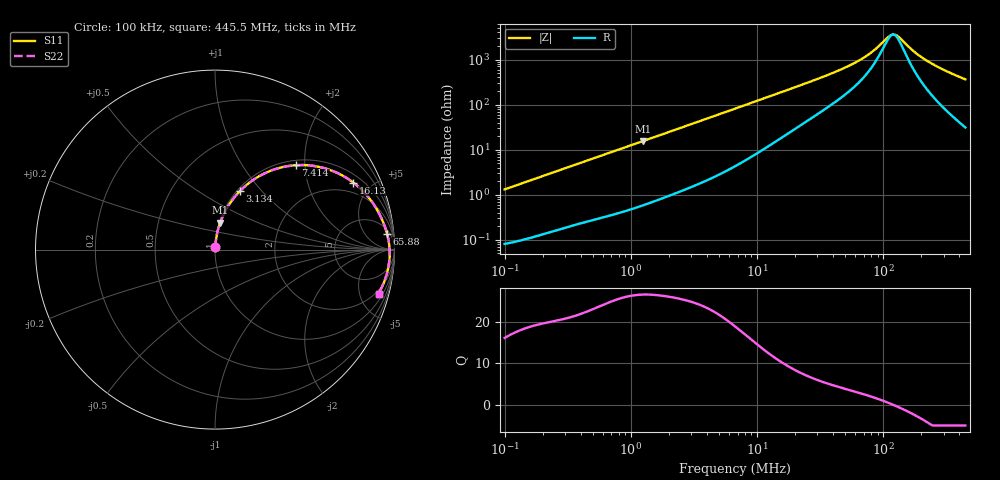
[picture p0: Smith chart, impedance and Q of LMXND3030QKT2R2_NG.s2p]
! LMXND3030QKT2R2_NG  S-PARAMETER MODEL  ( General Type )
! Model Generated by TAIYO YUDEN Corporation (http://www.ty-top.com)
! Version 1.0
! TAIYO YUDEN Control No. 191023NI43SB-FBB
! Copyright(c) 2019 TAIYO YUDEN CO.,LTD. All Rights Reserved.
! Product Description (link to TY-COMPAS)
! https://ds.yuden.co.jp/TYCOMPAS/or/detail?pn=LMXND3030QKT2R2MNG&u=M
! Products Name : Inductors
! Characteristics :
!  Inductance : 2.2 uH , SRF(min) : 64 MHz , DC Resistance(max) : 0.0696 Ohm
!  Rated Current : Saturation :1480 mA , Temp Rise : 1500 mA
!  Case Size : 3.0 x 3.0 / 0.118 x 0.118 [mm/inch] , Thickness : 1.5 / 0.059 [mm/inch]
!  (Conditions: Temperature = 25 degC , DC Bias Current/Voltage = 0A / 0V)
! External Node Assignments :
!  1  o---GGG---o  2
! GND o---------o GND
! Frequency Range : 0.1MHz  -  445.549718MHz  [ 402 STEP ]
# MHz S RI R 50
! Freq[MHz].  S11 Real  S11 Imag  S21 Real  S21 Imag  S12 Real  S12 Imag  S22 Real  S22 Imag
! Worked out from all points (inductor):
!   401 points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, 100 kHz to 445.5 MHz, reference 50 ohm
!   read as one part in series: L = 2.08 uH near 104.3 kHz
!   highest Q = 26.6 at 1.244 MHz (marker M1), where L = 1.98 uH
!   self-resonance near 119.2 MHz
!   S11 on the Smith chart (normalised r, x): 100 kHz: 1.00, +0.03; 3.134 MHz: 1.03, +0.77; 7.414 MHz: 1.10, +1.80; 16.13 MHz: 1.39, +3.90; 65.88 MHz: 8, +19; 445.5 MHz: 1.62, -7.22
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0.1  0.000985 0.0131  0.999 -0.0131  0.999 -0.0131  0.000985 0.0131
0.408498  0.00504 0.0516  0.995 -0.0516  0.995 -0.0516  0.00504 0.0516
1.243566  0.0287 0.1493  0.9713 -0.1493  0.9713 -0.1493  0.0287 0.1493
1.668708  0.0477 0.195  0.9523 -0.195  0.9523 -0.195  0.0477 0.195
3.133628  0.1381 0.3254  0.8619 -0.3254  0.8619 -0.3254  0.1381 0.3254
4.57349  0.2467 0.4094  0.7533 -0.4094  0.7533 -0.4094  0.2467 0.4094
6.81664  0.4116 0.4661  0.5884 -0.4661  0.5884 -0.4661  0.4116 0.4661
7.414114  0.4507 0.4703  0.5493 -0.4703  0.5493 -0.4703  0.4507 0.4703
10.59589  0.6152 0.452  0.3848 -0.452  0.3848 -0.452  0.6152 0.452
16.12806  0.7714 0.3728  0.2286 -0.3728  0.2286 -0.3728  0.7714 0.3728
27.26705  0.8856 0.2501  0.1144 -0.2501  0.1144 -0.2501  0.8856 0.2501
46.09929  0.9396 0.1462  0.0604 -0.1462  0.0604 -0.1462  0.9396 0.1462
65.88284  0.9589 0.0877  0.0411 -0.0877  0.0411 -0.0877  0.9589 0.0877
83.00742  0.9667 0.0529  0.0333 -0.0529  0.0333 -0.0529  0.9667 0.0529
111.3854  0.9723 0.00989  0.0277 -0.00989  0.0277 -0.00989  0.9723 0.00989
118.6301  0.9729 0.000658  0.0271 -0.000658  0.0271 -0.000658  0.9729 0.000658
126.3461  0.9732 -0.00864  0.0268 0.00864  0.0268 0.00864  0.9732 -0.00864
134.5639  0.9734 -0.018  0.0266 0.018  0.0266 0.018  0.9734 -0.018
173.1392  0.9717 -0.0569  0.0283 0.0569  0.0283 0.0569  0.9717 -0.0569
218.1424  0.9664 -0.0954  0.0336 0.0954  0.0336 0.0954  0.9664 -0.0954
305.2782  0.9498 -0.1592  0.0502 0.1592  0.0502 0.1592  0.9498 -0.1592
445.5497  0.9111 -0.2448  0.0889 0.2448  0.0889 0.2448  0.9111 -0.2448
